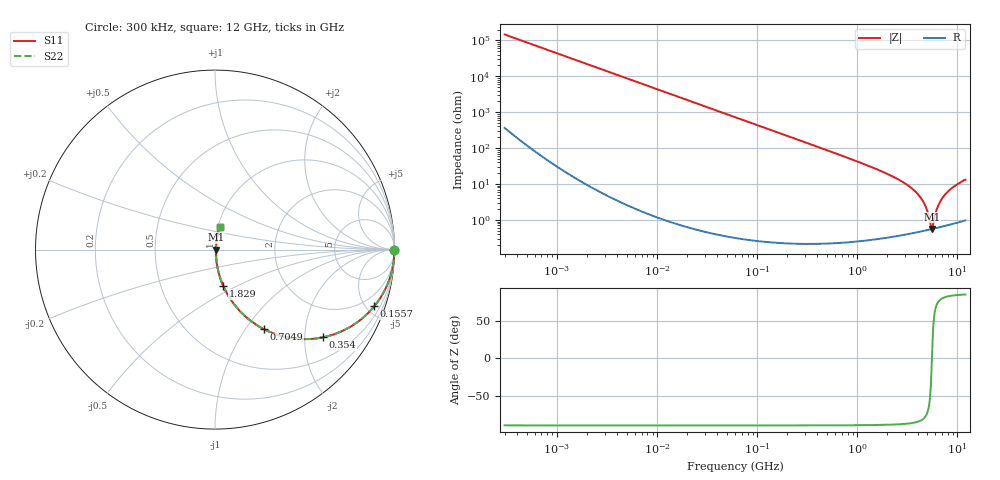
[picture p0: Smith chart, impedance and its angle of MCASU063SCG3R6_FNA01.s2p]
! MCASU063SCG3R6_FNA01  S-PARAMETER MODEL  ( Standard Model )
! Model Generated by TAIYO YUDEN Corporation (http://www.ty-top.com)
! Version 1.0
! TAIYO YUDEN Control No. 230609
! Copyright(c) 2023 TAIYO YUDEN CO.,LTD. All Rights Reserved.
! Product Description (link to TY-COMPAS)
! https://ds.yuden.co.jp/TYCOMPAS/or/detail?pn=MCASU063SCG3R6BFNA01&u=M
! Products Name : Multilayer Ceramic Capacitors
! Characteristics :
!  Capacitance : 3.6 [pF] , Rated Voltage : 50 [V] , TCC : CG / C0G
!  Case Size : 0.6 x 0.3 / 0.024 x 0.012 [mm/inch] , Thickness : 0.3 / 0.012 [mm/inch]
!  (Conditions: Temperature = 25 [degC] , DC Bias Voltage = 0 [V])
! External Node Assignments :
!  1  o---| |---o  2
! GND o---------o GND
! Frequency Range : 0.3MHz  -  12000MHz  [ 401 STEP ]
# MHZ S RI R 50
! Freq[MHz].  S11 Real  S11 Imag  S21 Real  S21 Imag  S12 Real  S12 Imag  S22 Real  S22 Imag
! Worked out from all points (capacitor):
!   401 points, 300 kHz to 12 GHz, reference 50 ohm
!   read as one part in series: C = 3.64 pF near 316.3 kHz
!   lowest |Z| = 558 mohm at 5.566 GHz (marker M1)
!   series resonance near 5.554 GHz, so ESL is about 230 pH
!   S11 on the Smith chart (normalised r, x): 300 kHz: open; 155.7 MHz: 1.00, -5.61; 354 MHz: 1.00, -2.46; 704.9 MHz: 1.00, -1.22; 1.829 GHz: 1.01, -0.43; 12 GHz: 1.02, +0.26
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0.3  1 -0.000687  2.19e-06 0.000687  2.19e-06 0.000687  1 -0.000687
1.769972  1 -0.00405  1.83e-05 0.00405  1.83e-05 0.00405  1 -0.00405
10.44266  0.9994 -0.0239  0.000577 0.0239  0.000577 0.0239  0.9994 -0.0239
60  0.9814 -0.1348  0.0186 0.1348  0.0186 0.1348  0.9814 -0.1348
155.7172  0.8869 -0.3162  0.1131 0.3162  0.1131 0.3162  0.8869 -0.3162
231.6935  0.7797 -0.4139  0.2203 0.4139  0.2203 0.4139  0.7797 -0.4139
353.9943  0.6016 -0.4887  0.3984 0.4887  0.3984 0.4887  0.6016 -0.4887
704.9044  0.2719 -0.4431  0.7281 0.4431  0.7281 0.4431  0.2719 -0.4431
1105.905  0.1276 -0.3302  0.8724 0.3302  0.8724 0.3302  0.1276 -0.3302
1829.429  0.0461 -0.2026  0.9539 0.2026  0.9539 0.2026  0.0461 -0.2026
2088.533  0.0343 -0.173  0.9657 0.173  0.9657 0.173  0.0343 -0.173
3107.553  0.0131 -0.0951  0.9869 0.0951  0.9869 0.0951  0.0131 -0.0951
4050.141  0.0071 -0.0502  0.9929 0.0502  0.9929 0.0502  0.0071 -0.0502
4623.766  0.00578 -0.029  0.9942 0.029  0.9942 0.029  0.00578 -0.029
4875.354  0.00552 -0.0207  0.9945 0.0207  0.9945 0.0207  0.00552 -0.0207
5278.635  0.00542 -0.00826  0.9946 0.00826  0.9946 0.00826  0.00542 -0.00826
5565.855  0.00554 0.000364  0.9945 -0.000364  0.9945 -0.000364  0.00554 0.000364
5715.274  0.00566 0.00492  0.9943 -0.00492  0.9943 -0.00492  0.00566 0.00492
6524.734  0.00685 0.0264  0.9932 -0.0264  0.9932 -0.0264  0.00685 0.0264
7254.098  0.00854 0.0438  0.9915 -0.0438  0.9915 -0.0438  0.00854 0.0438
8966.534  0.0139 0.0782  0.9861 -0.0782  0.9861 -0.0782  0.0139 0.0782
12000  0.0259 0.126  0.9741 -0.126  0.9741 -0.126  0.0259 0.126
